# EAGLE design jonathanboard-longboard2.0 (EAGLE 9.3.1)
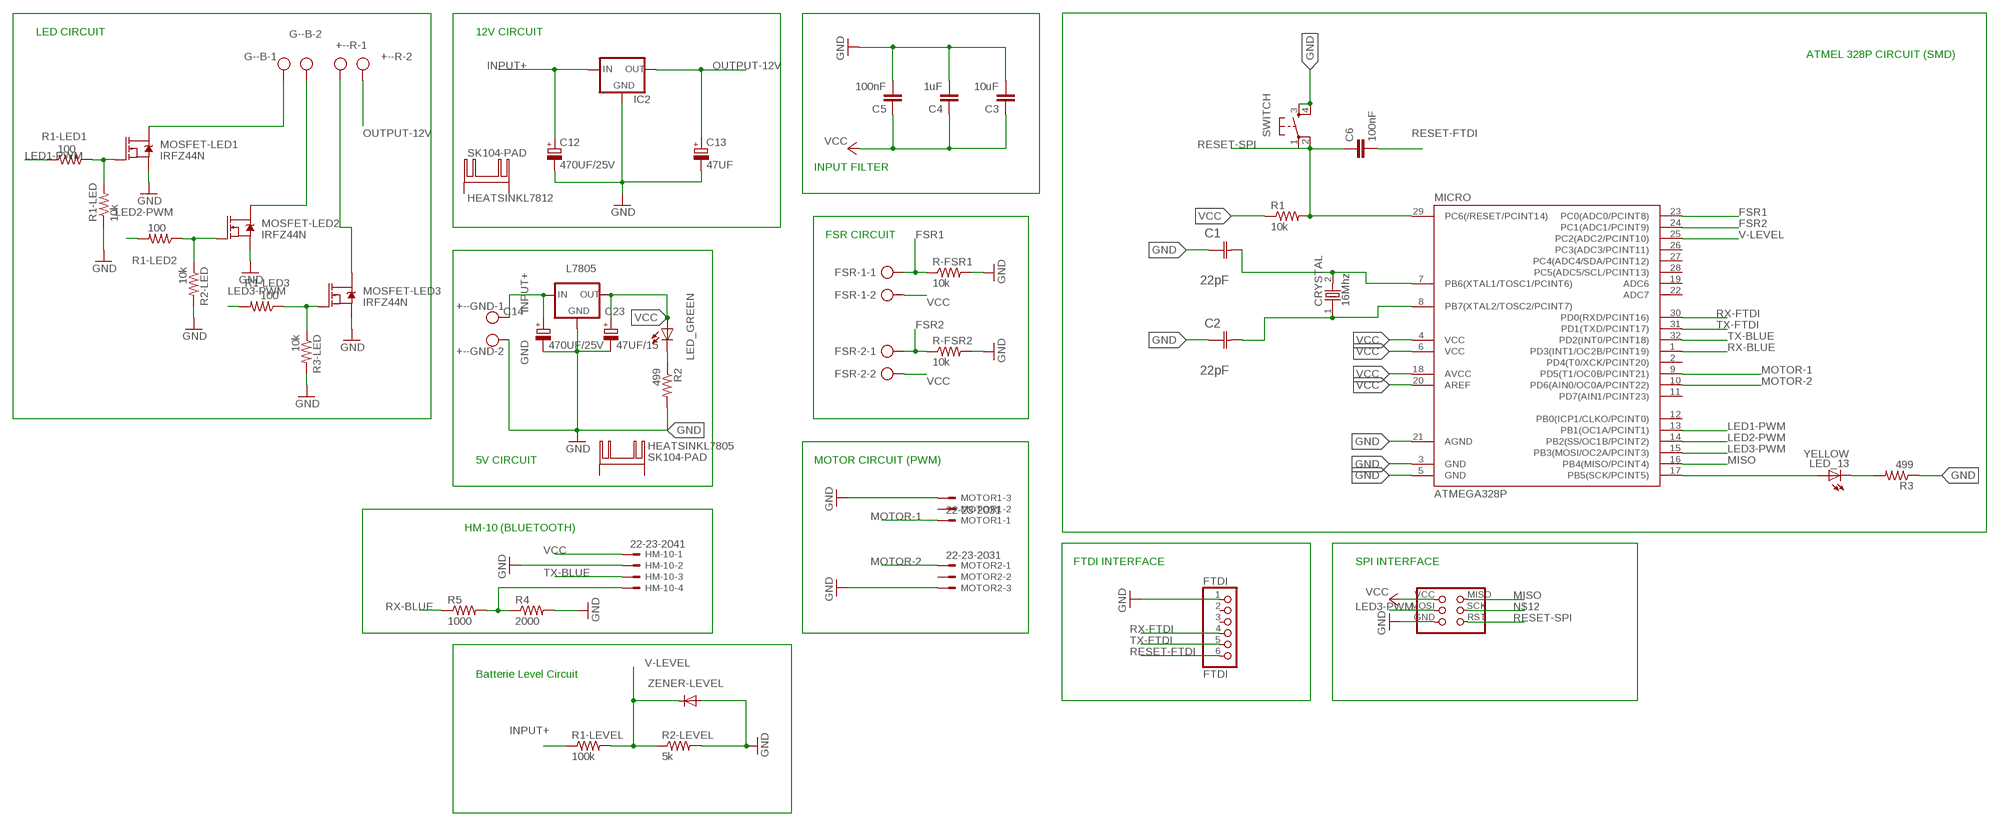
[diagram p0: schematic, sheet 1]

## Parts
+--GND  AK300/2  [AK300/2]
+--R  AK300/2  [AK300/2]
C1  22pF  0612ZC225MAT2A  [CAPC3216X178N]
C2  22pF  0612ZC225MAT2A  [CAPC3216X178N]
C3  10uF  CAP1206  [1206]
C4  1uF  CAP1206  [1206]
C5  100nF  CAP1206  [1206]
C6  100nF  CAP1206  [1206]
C12  470UF/25V  CPOL-EUE2.5-6  [E2,5-6]
C13  47UF  CPOL-EUE2.5-6  [E2,5-6]
C14  470UF/25V  CPOL-EUE2.5-6  [E2,5-6]
C23  47UF/15  CPOL-EUE2.5-6  [E2,5-6]
CRYSTAL  16Mhz  ABM3-8.000MHZ-D2Y-T  [XTAL500X320X130N]
FSR-1  AK300/2  [AK300/2]
FSR-2  AK300/2  [AK300/2]
FTDI  FTDI  PINHD-1X6_2.54-SMD-90°  [1X06SMD/90]
G--B  AK300/2  [AK300/2]
HEATSINKL7805  SK104-PAD  [SK104-PAD]
HEATSINKL7812  SK104-PAD  [SK104-PAD]
HM-10  22-23-2041  [22-23-2041]
IC1  L7805  [78XXS]
IC2  78XXS  [78XXS]
LED_13  YELLOW  LED1206  [1206]
LED_GREEN  LED1206  [1206]
MICRO  ATMEGA328P  ATMEGA48/88/168-AU  [TQFP32-08]
MOSFET-LED1  IRFZ44N  MOSFET-NCH-PSMN7R0  [TO-263/D2PAK]
MOSFET-LED2  IRFZ44N  MOSFET-NCH-PSMN7R0  [TO-263/D2PAK]
MOSFET-LED3  IRFZ44N  MOSFET-NCH-PSMN7R0  [TO-263/D2PAK]
MOTOR1  22-23-2031  [22-23-2031]
MOTOR2  22-23-2031  [22-23-2031]
R1  10k  RESISTOR1206  [1206]
R1-LED  10k  RESISTOR1206  [1206]
R1-LED1  100  RESISTOR1206  [1206]
R1-LED2  100  RESISTOR1206  [1206]
R1-LED3  100  RESISTOR1206  [1206]
R1-LEVEL  100k  RESISTOR1206  [1206]
R2  499  RESISTOR1206  [1206]
R2-LED  10k  RESISTOR1206  [1206]
R2-LEVEL  5k  RESISTOR1206  [1206]
R3  499  RESISTOR1206  [1206]
R3-LED  10k  RESISTOR1206  [1206]
R4  2000  RESISTOR1206  [1206]
R5  1000  RESISTOR1206  [1206]
R-FSR1  10k  RESISTOR1206  [1206]
R-FSR2  10k  RESISTOR1206  [1206]
SPI  2X3PINHEADER  [2X3PINHEADER]
SWITCH  6MM_SWITCH6MM_SWITCH  [6MM_SWITCH]
ZENER-LEVEL  DIODESOD123  [SOD123]

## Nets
FSR1: FSR-1.1 MICRO.23(PC0(ADC0/PCINT8)) R-FSR1.1
FSR2: FSR-2.1 MICRO.24(PC1(ADC1/PCINT9)) R-FSR2.1
GND: +--GND.2 C1.1(C1) C2.1(C1) C3.2 C4.2 C5.2 C12.- C13.- C14.- C23.- FTDI.1 HM-10.2 IC1.GND IC2.GND MICRO.3(GND) MICRO.5(GND) MICRO.21(AGND) MOSFET-LED1.3(S) MOSFET-LED2.3(S) MOSFET-LED3.3(S) MOTOR1.3 MOTOR2.3 R1-LED.1 R2-LED.2 R2-LEVEL.2 R2.2 R3-LED.2 R3.1 R4.2 R-FSR1.2 R-FSR2.2 SPI.GND SWITCH.3(S) SWITCH.4(S1) ZENER-LEVEL.ANODE(A)
INPUT+: +--GND.1 C12.+ C14.+ IC1.IN IC2.IN R1-LEVEL.1
LED1-PWM: MICRO.13(PB1(OC1A/PCINT1)) R1-LED1.2
LED2-PWM: MICRO.14(PB2(SS/OC1B/PCINT2)) R1-LED2.2
LED3-PWM: MICRO.15(PB3(MOSI/OC2A/PCINT3)) R1-LED3.2 SPI.MOSI
MISO: MICRO.16(PB4(MISO/PCINT4)) SPI.MISO
MOTOR-1: MICRO.9(PD5(T1/OC0B/PCINT21)) MOTOR1.1
MOTOR-2: MICRO.10(PD6(AIN0/OC0A/PCINT22)) MOTOR2.1
N$5: MOSFET-LED1.1(G) R1-LED1.1 R1-LED.2
N$6: MOSFET-LED2.1(G) R1-LED2.1 R2-LED.1
N$10: MOSFET-LED3.1(G) R1-LED3.1 R3-LED.1
N$11: HM-10.4 R4.1 R5.2
N$12: LED_13.1(A) MICRO.17(PB5(SCK/PCINT5)) SPI.SCK
N$19: C1.2(C2) CRYSTAL.2 MICRO.7(PB6(XTAL1/TOSC1/PCINT6))
N$21: C2.2(C2) CRYSTAL.1 MICRO.8(PB7(XTAL2/TOSC2/PCINT7))
N$26: LED_GREEN.2(C) R2.1
N$27: LED_13.2(C) R3.2
N$29: G--B.1 MOSFET-LED1.2(D)
N$30: G--B.2 MOSFET-LED2.2(D)
N$31: +--R.1 MOSFET-LED3.2(D)
OUTPUT-12V: +--R.2 C13.+ IC2.OUT
RESET-FTDI: C6.2 FTDI.6
RESET-SPI: C6.1 MICRO.29(PC6(/RESET/PCINT14)) R1.2 SPI.RST SWITCH.1(P) SWITCH.2(P1)
RX-BLUE: MICRO.1(PD3(INT1/OC2B/PCINT19)) R5.1
RX-FTDI: FTDI.4 MICRO.30(PD0(RXD/PCINT16))
TX-BLUE: HM-10.3 MICRO.32(PD2(INT0/PCINT18))
TX-FTDI: FTDI.5 MICRO.31(PD1(TXD/PCINT17))
V-LEVEL: MICRO.25(PC2(ADC2/PCINT10)) R1-LEVEL.2 R2-LEVEL.1 ZENER-LEVEL.CATHODE(C)
VCC: C3.1 C4.1 C5.1 C23.+ FSR-1.2 FSR-2.2 HM-10.1 IC1.OUT LED_GREEN.1(A) MICRO.4(VCC) MICRO.6(VCC) MICRO.18(AVCC) MICRO.20(AREF) R1.1 SPI.VCC
Unconnected: FTDI.2 FTDI.3 HEATSINKL7805.K1(K) HEATSINKL7805.K2(K) HEATSINKL7812.K1(K) HEATSINKL7812.K2(K) MICRO.2(PD4(T0/XCK/PCINT20)) MICRO.11(PD7(AIN1/PCINT23)) MICRO.12(PB0(ICP1/CLKO/PCINT0)) MICRO.19(ADC6) MICRO.22(ADC7) MICRO.26(PC3(ADC3/PCINT11)) MICRO.27(PC4(ADC4/SDA/PCINT12)) MICRO.28(PC5(ADC5/SCL/PCINT13)) MOTOR1.2 MOTOR2.2

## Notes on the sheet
- LED CIRCUIT | 12V CIRCUIT
- ATMEL 328P CIRCUIT (SMD)
- INPUT FILTER
- FSR CIRCUIT
- 5V CIRCUIT | MOTOR CIRCUIT (PWM)
- HM-10 (BLUETOOTH)
- FTDI INTERFACE | SPI INTERFACE
- Batterie Level Circuit

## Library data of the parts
+--GND +--R FSR-1 FSR-2 G--B = con-ptr500:AK300/2: CONNECTOR; OC_FARNELL: unknown; OC_NEWARK: unknown
C1 C2 = AVX_By_element14_Batch_1:0612ZC225MAT2A: Capacitor 1206; MPN: 0612ZC225MAT2A; OC_FARNELL: -; OC_NEWARK: 12N3209; SUPPLIER: AVX; TOLERANCE: ±20%; VALUE: 2.2µF; VOLTAGERATING: 10V
C3-C6 = 01_SparkFun:CAP: Capacitor
C12-C14 C23 = rcl:CPOL-EU: POLARIZED CAPACITOR, European symbol; SPICEPREFIX: C
CRYSTAL = ABM3-8.000MHZ-D2Y-T:ABM3-8.000MHZ-D2Y-T: Crystals 12MHz 18pF 30ppm -40C +85C; AVAILABILITY: Unavailable; DESCRIPTION: Crystal 8MHz Ø·Â¢Ø¢Â±20ppm _Tol_ Ø·Â¢Ø¢Â±30ppm _Stability_ 18pF FUND 500Ohm 2-Pin CSMD T/R; MF: Abracon; MP: ABM3-8.000MHZ-D2Y-T; PACKAGE: SMD-2 Abracon; PRICE: None
FTDI = pinhead-1:PINHD-1X6: PIN HEADER
HEATSINKL7805 HEATSINKL7812 = heatsink-jonathan:SK104-PAD: HEATSINK
HM-10 = con-molex:22-23-2041: .100" (2.54mm) Center Header - 4 Pin; MF: MOLEX; MPN: 22-23-2041; OC_FARNELL: 1462920; OC_NEWARK: 38C0355
IC1 = L7805:L7805: ICP001; AVAILABILITY: Unavailable; MF: STMicroelectronics; MP: L7805; PACKAGE: None; PRICE: None
IC2 = v-reg:78XXS: VOLTAGE REGULATOR
LED_13 LED_GREEN = 01_FAB_Hello:LED
MICRO = atmega8:ATMEGA48/88/168
MOSFET-LED1-MOSFET-LED3 = SparkFun-DiscreteSemi:MOSFET-NCH: N-channel MOSFETs Voltage controlled devices that allow control of high current outputs. SparkFun Products: SparkFun OpenScale SparkFun Digital Sandbox SparkFun Monster Moto Shield SparkFun MOSFET Power Controller; PROD_ID: TRANS-12437; VALUE: 100A/100V/6.8mΩ
MOTOR1 MOTOR2 = con-molex:22-23-2031: .100" (2.54mm) Center Header - 3 Pin; MF: MOLEX; MPN: 22-23-2031; OC_FARNELL: 1462950; OC_NEWARK: 30C0862
R1 R1-LED R1-LED1-R1-LED3 R1-LEVEL R2 R2-LED R2-LEVEL R3 R3-LED R4 R5 R-FSR1 R-FSR2 = 01_SparkFun:RESISTOR: Resistor
SPI = myFab:2X3PINHEADER: PIN HEADER
SWITCH = 01_FAB_Hello:6MM_SWITCH: OMRON SWITCH
ZENER-LEVEL = fab:DIODE: DIODE

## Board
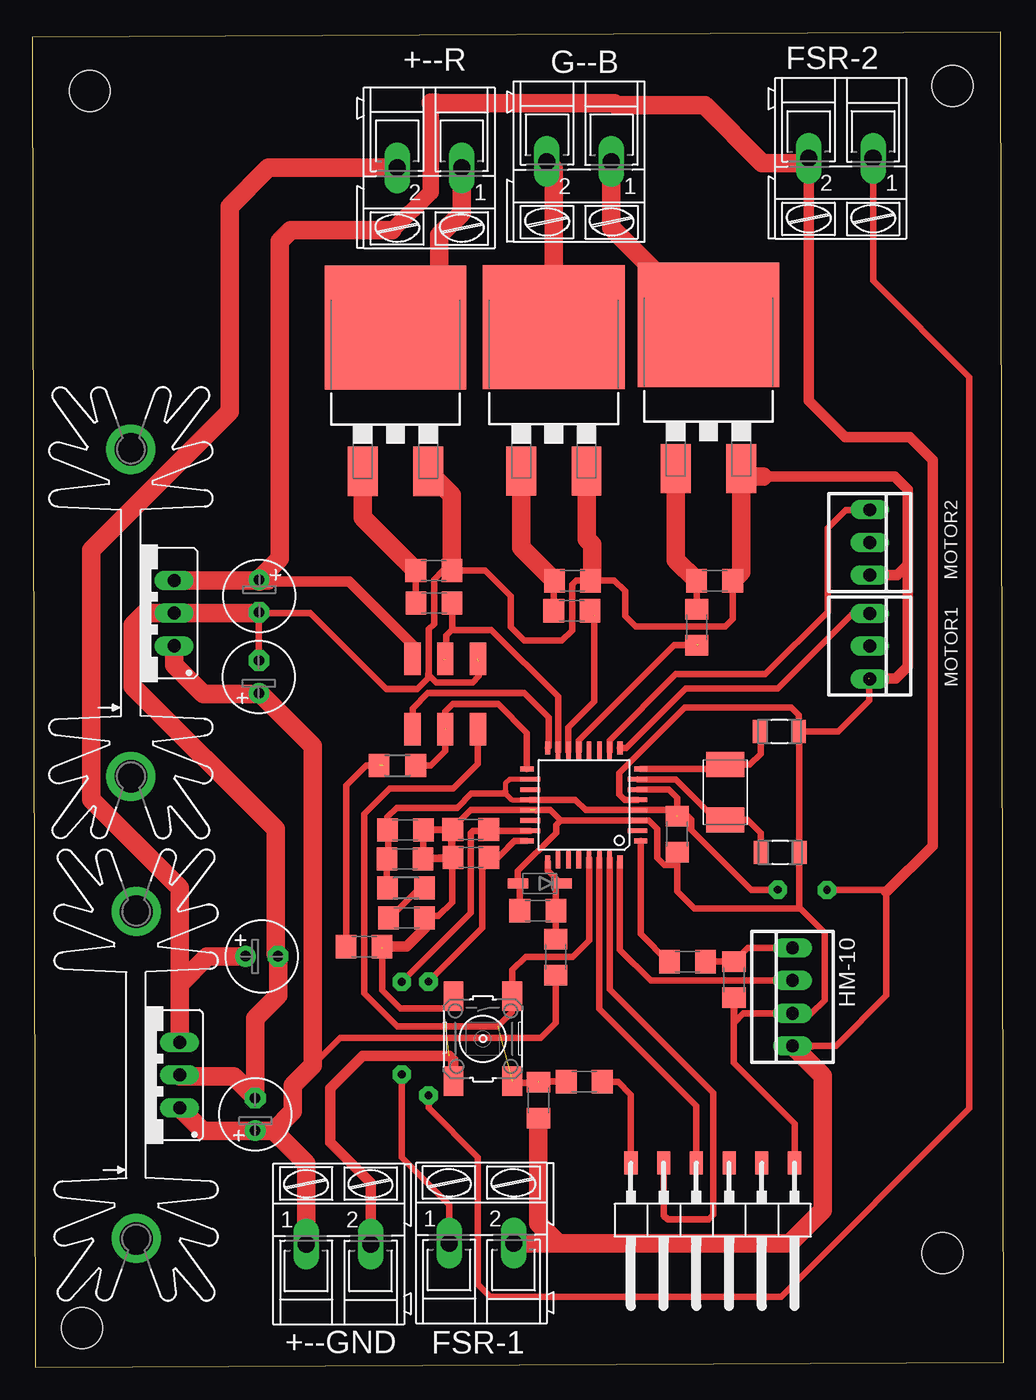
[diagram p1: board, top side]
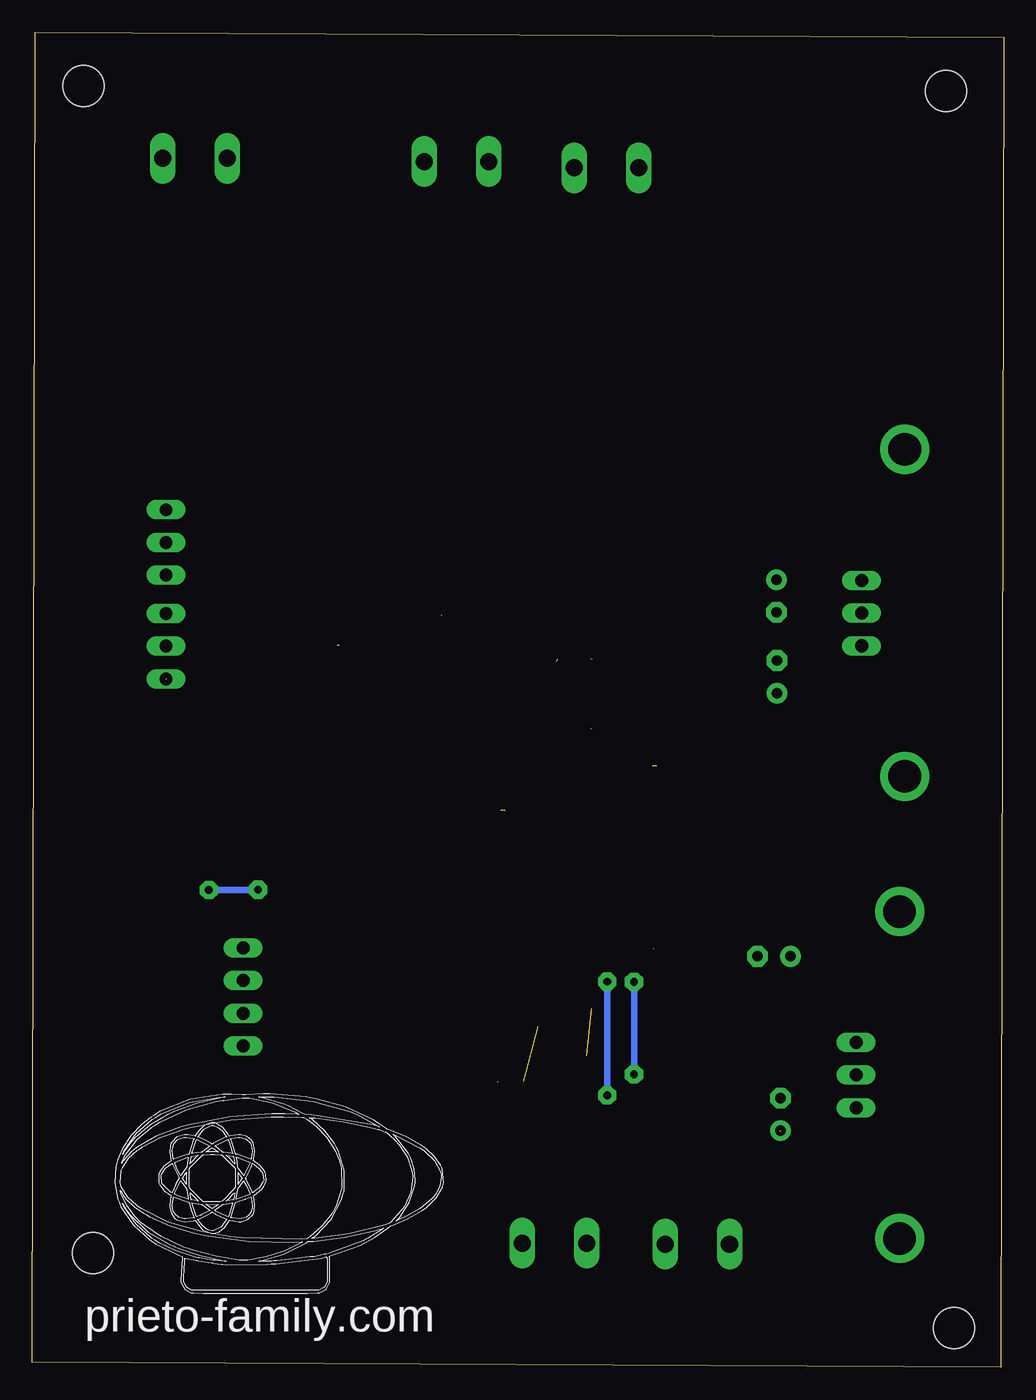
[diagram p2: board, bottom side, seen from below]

Size 75.44 x 103.73 mm. Coordinates in mm from the lower left corner, seen from the top.
Outline: 0.23,0 75.44,0.41 75.21,103.73 0,103.33 0.23,0
Copper layers (1*16): Top 0.035mm / dielectric 1.5mm / Bottom 0.035mm
Design rules "default": minimum track width 6mil, minimum drill 0.35mm, track to track 6mil, track to pad 6mil, pad to pad 6mil, via to via 6mil, smd to smd 6mil, copper to edge 40mil, drill to drill 6mil, minimum pad ring 10mil, minimum via ring 8mil, stop-mask expansion 4mil, vias tented up to drill 0mil, thermal gap 10mil
Holes 3.2 mm at 4.47,99.16 71.48,99.54 3.86,3.05 70.71,8.86

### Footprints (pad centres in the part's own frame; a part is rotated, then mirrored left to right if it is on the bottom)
AK300/2 = drill 1.321 long: 1 -2.515,0; 2 2.489,0
CAPC3216X178N = smd 1.118 x 1.803: 1 -1.499,0; 2 1.499,0
1206 = smd 1.6 x 1.8: 1 -1.4,0; 2 1.4,0
E2,5-6 = drill 0.813 pad 1.6: + -1.27,0 | drill 0.813 pad 1.6 octagon: - 1.27,0
XTAL500X320X130N = smd 1.95 x 2.95: 1 -2.15,0; 2 2.15,0
1X06SMD/90 = smd 1.016 x 1.778: 1 -1.27,-5.08; 2 1.27,-5.08; 3 3.81,-5.08; 4 6.35,-5.08; 5 8.89,-5.08; 6 11.43,-5.08
SK104-PAD = drill 2.54 pad 3.81: K1 -12.7,-0.762; K2 12.7,-0.762
22-23-2041 = drill 1 long: 1 -3.81,0; 2 -1.27,0; 3 1.27,0; 4 3.81,0
78XXS = drill 1.016 long: GND 0,-2.54; IN -2.54,-2.54; OUT 2.54,-2.54
1206' = smd 1.6 x 1.803: 1 -1.422,0; 2 1.422,0
TQFP32-08 = smd 1.016 x 0.406: 1 -4.42,2.8; 8 -4.42,-2.8; 17 4.42,-2.8; 24 4.42,2.8 | smd 1.524 x 0.356: 2 -4.166,2; 3 -4.166,1.2; 4 -4.166,0.4; 5 -4.166,-0.4; 6 -4.166,-1.2; 7 -4.166,-2; 18 4.166,-2; 19 4.166,-1.2; 20 4.166,-0.4; 21 4.166,0.4; 22 4.166,1.2; 23 4.166,2 | smd 0.406 x 1.016: 9 -2.8,-4.42; 16 2.8,-4.42; 25 2.8,4.42; 32 -2.8,4.42 | smd 0.356 x 1.524: 10 -2,-4.166; 11 -1.2,-4.166; 12 -0.4,-4.166; 13 0.4,-4.166; 14 1.2,-4.166; 15 2,-4.166; 26 2,4.166; 27 1.2,4.166; 28 0.4,4.166; 29 -0.4,4.166; 30 -1.2,4.166; 31 -2,4.166
TO-263/D2PAK = smd 2.32 x 3.81: 1 -2.54,-7.045; 3 2.54,-7.045 | smd 11 x 9.65: 2 0,4.125
22-23-2031 = drill 1 long: 1 -2.54,0; 2 0,0; 3 2.54,0
2X3PINHEADER = smd 2.54 x 1.27: GND -2.54,2.54; MISO 2.92,-2.54; MOSI -2.54,0; RST 2.92,2.54; SCK 2.92,0; VCC -2.54,-2.54
6MM_SWITCH = smd 2.286 x 1.524: 1 -3.302,2.286; 2 3.302,2.286; 3 -3.302,-2.286; 4 3.302,-2.286
SOD123 = smd 1.6 x 0.8: ANODE 1.7,0; CATHODE -1.7,0

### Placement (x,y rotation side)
+--GND  23.8,9.58 0 top
+--R  30.84,93.19 180 top
C1  58.09,40.01 180 top
C2  58.04,49.4 180 top
C3  28.96,39.5 0 top
C4  50.09,41.43 270 top
C5  28.98,41.76 0 top
C6  42.88,22.2 0 top
C12  17.6,53.64 90 top
C13  17.83,31.93 0 top
C14  17.32,19.66 90 top
C23  17.63,59.92 270 top
CRYSTAL  53.82,44.68 270 top
FSR-1  34.9,9.65 0 top
FSR-2  62.79,93.93 180 top
FTDI  57.94,10.79 180 top
G--B  42.47,93.68 180 top
HEATSINKL7805  7.32,22.71 90 top
HEATSINKL7812  6.91,58.62 90 top
HM-10  59.05,28.78 90 top
IC1  8.48,58.6 90 top
IC2  8.92,22.71 90 top
LED_13  YELLOW  [1206']  28.37,46.76 180 top
LED_GREEN  [1206']  29.03,37.24 0 top
MICRO  42.85,43.69 180 top
MOSFET-LED1  52.53,76.86 0 top
MOSFET-LED2  40.51,76.68 0 top
MOSFET-LED3  28.22,76.66 0 top
MOTOR1  65.05,56.03 270 top
MOTOR2  65.05,64.08 270 top
R1  39.32,20.75 90 top
R1-LED  53.01,61.11 180 top
R1-LED1  51.61,57.51 270 top
R1-LED2  41.91,58.78 0 top
R1-LED3  31.22,59.39 0 top
R1-LEVEL  40.67,31.88 90 top
R2  29.08,34.92 0 top
R2-LED  41.96,61.11 0 top
R2-LEVEL  39.27,35.48 180 top
R3  25.78,32.69 180 top
R3-LED  31.19,61.9 0 top
R4  54.51,30.12 270 top
R5  50.9,31.52 0 top
R-FSR1  34.06,41.78 180 top
R-FSR2  34.09,39.62 180 top
SPI  32.08,52.5 270 top
SWITCH  35,25.53 270 top
ZENER-LEVEL  39.42,37.59 180 top

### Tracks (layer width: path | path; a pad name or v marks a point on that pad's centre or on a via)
FSR1  (via drill 0.6 pad 1.42)
  Top 0.508: MICRO.23 35.56,41.69 | 35.56,41.69 R-FSR1.1 | 35.56,41.69 34.22,41.69 34.06,41.53 34.06,35.31 v28.7,29.95 | v28.7,22.76 28.7,16.31 32.38,12.62 FSR-1.1
  Bottom 0.508: v28.7,29.95 v28.7,22.76
FSR2  (via drill 0.6 pad 1.42)
  Top 0.508: 36.3,39.73 36.19,39.62 35.69,39.62 35.66,39.6 35.51,39.6 R-FSR2.1 | 35.53,39.45 35.76,39.67 36.27,39.67 37.48,40.89 MICRO.24 37.46,40.89 36.3,39.73 | 36.3,39.73 35.97,39.73 34.95,38.71 34.95,34.14 v30.78,29.97 | v30.78,21.13 30.78,20.14 34.62,16.31 34.62,6.45 35.59,5.49 58.17,5.49 72.8,20.12 72.8,76.94 65.3,84.43 FSR-2.1
  Bottom 0.508: v30.78,29.97 v30.78,21.13
GND  (6 unrouted)
  Top 0.508: MICRO.21 40.25,43.29 41.05,42.49 | 41.05,42.49 MICRO.3 47.89,42.49 48.54,41.83 48.54,39.57 49.1,39.01 50.03,39.01 C4.2 50.09,36.98 51.41,35.66 59.64,35.66 | C1.1 59.59,49.33 | C2.1 59.59,49.35 59.59,49.33 | 59.61,40.03 C1.1 | R1-LED.1 54.41,58.14 53.82,57.56 46.86,57.56 46.05,58.37 46.05,60.3 45.21,61.14 43.39,61.14 R2-LED.2 43.34,61.14 42.27,61.14 41.94,60.81 41.94,57.25 41.15,56.46 38.2,56.46 37.16,57.51 37.16,59.92 35.18,61.9 R3-LED.2 32.57,61.92 31.93,61.92 31.22,61.21 31.22,57.76 30.81,57.35 30.81,53.8 | 59.59,49.33 59.41,49.15 | C1.1 59.59,35.71 59.64,35.66 | C2.1 62.61,49.4 65.02,51.82 65.02,53.47 MOTOR1.3 | 59.56,49.43 C2.1 | R2-LEVEL.2 37.87,37.44 ZENER-LEVEL.ANODE 37.72,38.56 40.69,41.53 40.69,42.14 41.05,42.49 | SPI.GND 34.62,53.97 | 30.81,53.8 30.76,53.85 30.76,53.64 30.81,53.59 29.92,52.7 27.51,52.7 21.59,58.62 17.6,58.62 C12.- | 30.81,53.8 31.39,53.21 34.21,53.21 34.7,53.7 34.7,54.84 34.87,55.02 | FTDI.1 59.21,18.92 54.48,23.65 54.48,28.7 R4.2 54.46,28.67 54.46,28.63 54.51,28.57 54.51,26.77 55.24,27.51 HM-10.2 | R2.2 30.33,34.92 | 32.61,39.34 32.61,36.12 31.55,35.05 30.45,35.05 30.33,34.92 | 32.61,39.34 32.54,39.42 32.54,39.5 | C3.2 31.65,39.62 R-FSR2.2 32.53,42.01 32.61,42.09 32.61,41.91 | C3.2 30.36,41.73 C5.2 | R-FSR1.2 30.41,41.78 C5.2 | C3.2 32.54,39.5 | C5.2 32.51,41.76 32.59,41.68 | 32.54,39.5 32.54,41.86 32.59,41.91 32.59,41.76 | 32.61,39.34 32.61,41.86 34.06,43.31 39.07,43.31 39.12,43.26 | MICRO.5 46.03,44.09 45.59,44.53 45.59,46.18 50.7,51.28 58.95,51.28 59.54,50.7 59.54,49.61 59.39,49.45 59.44,49.4 C2.1 | 30.33,34.92 30.2,34.8 | SWITCH.3 32.72,28.63 31.98,27.89 28.6,27.89 27.2,29.29 27.2,32.54 27.48,32.82
  Top 0.508: 59,27.53 59.05,27.48 60.5,27.48 61.54,28.52 61.54,33.76 59.64,35.66
  Top 0.813: 56.79,69.21 67.01,69.21 68.02,68.2 | 68.02,68.2 68.02,54.46 67.08,53.52 64.97,53.52 64.95,53.49 | MOTOR2.3 67.18,61.54 68,62.36 68,68.17 68.02,68.2 | R2.2 30.48,34.09 29.08,32.69 27.28,32.69 27.15,32.56 27.15,32.66 R3.1 | +--GND.2 26.29,14.33 23.14,17.47 23.14,21.67 25.68,24.21 32.38,24.21 32.72,23.88 SWITCH.4
  Top 1.422: IC2.GND 11.46,22.61 15.64,22.61 C14.- 17.32,27.1 19.1,28.88 C13.- 18.9,32.13 18.9,41.83 7.82,52.91 7.82,57.68 8.74,58.6 IC1.GND 17.58,58.6 17.6,58.62 C23.- | 56.79,69.21 55.67,69.21 MOSFET-LED1.3 55.07,61.77 R1-LED.1 | MOSFET-LED2.3 43.05,64.36 43.51,63.91 43.51,61.26 R2-LED.2 | MOSFET-LED3.3 32.59,67.78 R3-LED.2
INPUT+  (1 unrouted)
  Top 0.508: R1-LEVEL.1 40.67,26.75 39.5,25.58 23.93,25.58 21.79,23.44
  Top 1.422: IC1.IN 11.02,54.58 13.28,52.32 17.55,52.32 | 17.55,52.32 C12.+ | C14.+ 13.23,18.39 IC2.IN | 17.55,52.32 17.75,52.32 21.79,48.29 21.79,23.44 20.24,21.89 20.24,19.89 18.75,18.39 | 18.75,18.39 18.72,18.39 | 17.37,18.36 17.4,18.39 18.72,18.39 | +--GND.1 21.29,15.85 18.75,18.39 | 18.72,18.39 18.75,18.41
LED1-PWM  (1 unrouted)
  Top 0.508: 51.59,56.08 R1-LED1.2 | MICRO.13 42.45,48.7 49.89,56.13 51.74,56.13 51.82,56.21
LED2-PWM  (1 unrouted)
  Top 0.508: 43.66,58.42 R1-LED2.2 | MICRO.14 41.65,49.73 43.64,51.71 43.64,58.42 43.71,58.5
LED3-PWM  (1 unrouted)
  Top 0.508: MICRO.15 40.85,52.11 35.66,57.3 32.72,57.3 | 32.72,57.3 32.59,57.3 32.16,56.87 32.16,55.22 31.93,54.99 | R1-LED3.2 32.62,57.4 32.72,57.3
MISO
  Top 0.508: SPI.MISO 29.54,51.18 30.73,52.37 38.23,52.37 40.13,50.47 40.13,48.19 MICRO.16
MOTOR-1
  Top 0.508: MICRO.9 46.13,48.11 50.77,52.76 57.91,52.76 63.73,58.57 64.97,58.57 65.02,58.52 65.02,58.55 MOTOR1.1
MOTOR-2
  Top 0.508: MICRO.10 44.85,48.71 49.99,53.85 56.95,53.85 61.77,58.67 61.77,65.2 63.17,66.6 65.05,66.6 MOTOR2.1
N$5
  Top 0.508: R1-LED.2 R1-LED1.1
  Top 1.422: MOSFET-LED1.1 49.99,62.73 R1-LED.2
N$6
  Top 0.508: R1-LED2.1 40.51,61.06 R2-LED.1 39.65,62.02
  Top 1.422: MOSFET-LED2.1 37.97,63.7 R2-LED.1
N$10
  Top 0.508: 28.57,63.12 R3-LED.1 29.79,59.41 R1-LED3.1
  Top 1.422: MOSFET-LED3.1 25.68,66.01 R3-LED.1
N$11
  Top 0.508: R5.2 R4.1 55.57,32.59 HM-10.4
N$12  (1 unrouted)
  Top 0.508: SPI.SCK 32.08,50.95 32.66,51.54 36.19,51.54 38.43,49.3 MICRO.17 | LED_13.1 30.94,46.76 32.08,47.9 32.08,49.63 32.16,49.71
N$19
  Top 0.508: MICRO.7 49.98,45.69 53.14,42.53 CRYSTAL.2 53.82,42.49 53.85,42.52 55.58,42.52 56.59,41.5 C1.2
N$21
  Top 0.508: MICRO.8 53.48,46.49 CRYSTAL.1 55.74,46.83 56.57,47.65 56.57,49.35 56.64,49.43 56.57,49.43 C2.2
N$26
  Top 0.508: R2.1 27.79,34.92 29.79,36.93 30.15,36.93 LED_GREEN.2
N$27  (1 unrouted)
  Top 0.508: R3.2 24.38,45.21 25.93,46.76 27.28,46.76 27.33,46.81
N$29
  Top 1.422: MOSFET-LED1.2 44.98,88.53 G--B.1
N$30
  Top 1.422: MOSFET-LED2.2 40.51,93.14 G--B.2
N$31
  Top 1.422: MOSFET-LED3.2 31.62,84.19 31.62,87.96 33.35,89.69 +--R.1
OUTPUT-12V
  Top 1.422: IC2.OUT 11.46,29.77 | 11.46,29.77 11.46,37.26 4.6,44.12 4.6,63.5 15.34,74.24 15.34,90.2 18.34,93.19 +--R.2 | C13.+ 13.61,31.93 11.46,29.77
RESET-FTDI
  Top 0.508: FTDI.6 46.51,21.18 45.52,22.17 44.3,22.17 C6.2
RESET-SPI  (2 unrouted)
  Top 0.508: 37.77,28.83 SWITCH.1 37.26,28.8 37.26,28.14 | MICRO.29 43.25,34.32 43.26,34.32 43.26,33.17 41.99,31.9 38.33,31.9 37.29,30.86 37.29,28.12 37.26,28.14 | C6.1 39.29,22.2 39.19,22.1 37.41,22.1 SWITCH.2 | SPI.RST 34.62,46.89 32.69,44.96 27.76,44.96 25.78,42.98 25.78,29.06 28.35,26.49 36.17,26.49 37.26,27.58 37.26,28.14
RX-BLUE
  Top 0.508: MICRO.1 47.27,33.65 49.45,31.47 R5.1
RX-FTDI
  Top 0.508: MICRO.30 44.05,27.86 51.59,20.32 FTDI.4
TX-BLUE
  Top 0.508: MICRO.32 45.65,32.43 48.03,30.05 HM-10.3 59.11,30.05
TX-FTDI
  Top 0.508: MICRO.31 44.85,29.34 52.88,21.31 52.88,11.84 52.53,11.48 49.35,11.48 49.05,11.79 FTDI.5
V-LEVEL
  Top 0.508: MICRO.25 40.05,38.61 40.74,37.92 | 40.74,37.92 41.07,37.59 ZENER-LEVEL.CATHODE | 40.74,37.92 40.67,37.85 R2-LEVEL.1 R1-LEVEL.2
VCC  (via drill 0.6 pad 1.42)  (2 unrouted)
  Top 0.406: 38.71,44.09 37.26,44.09 36.75,44.6 36.75,44.75 36.75,45.36 37.08,45.69 MICRO.18
  Top 0.508: MICRO.20 38.71,44.09 42.19,44.09 43,43.29 MICRO.4 49.63,43.29 C4.1 | v61.72,37.08 66.19,37.08 66.34,36.93 66.34,28.88 62.43,24.97 60.17,24.97 | 49.68,42.39 C4.1 50.09,44.22 49.42,44.89 MICRO.6 | 60.2,24.94 59.03,24.94 | LED_GREEN.1 27.56,37.29 C3.1 27.64,39.5 27.64,41.7 C5.1 27.58,42.74 28.3,43.46 32.99,43.46 34.11,44.58 36.58,44.58 36.75,44.75 | v57.91,37.11 55.83,37.11 51.21,41.73 51.21,42.57 50.93,42.85 50.06,42.85 | 60.17,24.97 58.9,24.97 | 60.6,24.94 60.2,24.94 | 60.2,24.94 60.17,24.97
  Top 0.813: 59.03,24.94 HM-10.1 | 66.34,36.93 69.93,40.51 69.93,70.48 68.15,72.26 63.14,72.26 60.3,75.11 60.3,93.55 FSR-2.2 60.3,94.03 | 17.63,61.04 24.61,61.04 29.62,56.03 29.62,55.12 SPI.VCC
  Top 1.27: 30.94,98.26 30.94,91.31 27.97,88.34
  Top 1.422: 17.53,61.14 17.63,61.04 | FSR-1.2 40.87,9.65 | 40.87,9.65 58.85,9.65 61.39,12.19 61.39,22.63 HM-10.1 | R1.1 39.32,11.2 40.87,9.65 | 17.58,61.14 18.31,61.14 | IC1.OUT 17.53,61.14 | 17.53,61.14 17.58,61.14 | 17.58,61.14 C23.+ | 60.3,93.55 56.72,93.55 52.22,98.04 45.36,98.04 45.21,98.2 31.5,98.2 31.43,98.26 30.94,98.26 | 27.97,88.34 20.09,88.34 19.23,87.48 19.23,62.84 17.53,61.14
  Bottom 0.508: v61.72,37.08 57.94,37.08 v57.91,37.11

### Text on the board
bPlace: prieto-family.com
